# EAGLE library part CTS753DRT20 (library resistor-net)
Network Resistor CTS 753 Series Leadless Surface Mount Source: http://www.ctscorp.com/components/Datasheets/753.pdf Distributor: Digi Key
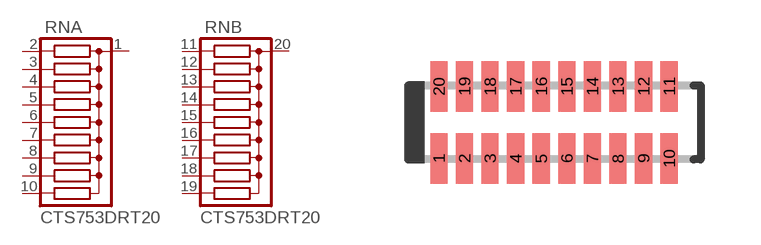
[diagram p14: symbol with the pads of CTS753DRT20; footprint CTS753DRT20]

Designator prefix RN; gates A=RN1X9 B=RN1X9

## CTS753DRT20 (OC_FARNELL: unknown; OC_NEWARK: unknown)  [CTS753DRT20]
1  A:C  pas
2  A:1  pas
3  A:2  pas
4  A:3  pas
5  A:4  pas
6  A:5  pas
7  A:6  pas
8  A:7  pas
9  A:8  pas
10  A:9  pas
11  B:1  pas
12  B:2  pas
13  B:3  pas
14  B:4  pas
15  B:5  pas
16  B:6  pas
17  B:7  pas
18  B:8  pas
19  B:9  pas
20  B:C  pas

## Footprint CTS753DRT20 (pad centres in mm)
Network Resistor Leadless Surface Mount Series 753 Source: http://www.ctscorp.com/components/Datasheets/753.pdf
smd 0.43 x 1.27: 1 -2.88,-0.9; 2 -2.24,-0.9; 3 -1.6,-0.9; 4 -0.96,-0.9; 5 -0.32,-0.9; 6 0.32,-0.9; 7 0.96,-0.9; 8 1.6,-0.9; 9 2.24,-0.9; 10 2.88,-0.9; 11 2.88,0.9; 12 2.24,0.9; 13 1.6,0.9; 14 0.96,0.9; 15 0.32,0.9; 16 -0.32,0.9; 17 -0.96,0.9; 18 -1.6,0.9; 19 -2.24,0.9; 20 -2.88,0.9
